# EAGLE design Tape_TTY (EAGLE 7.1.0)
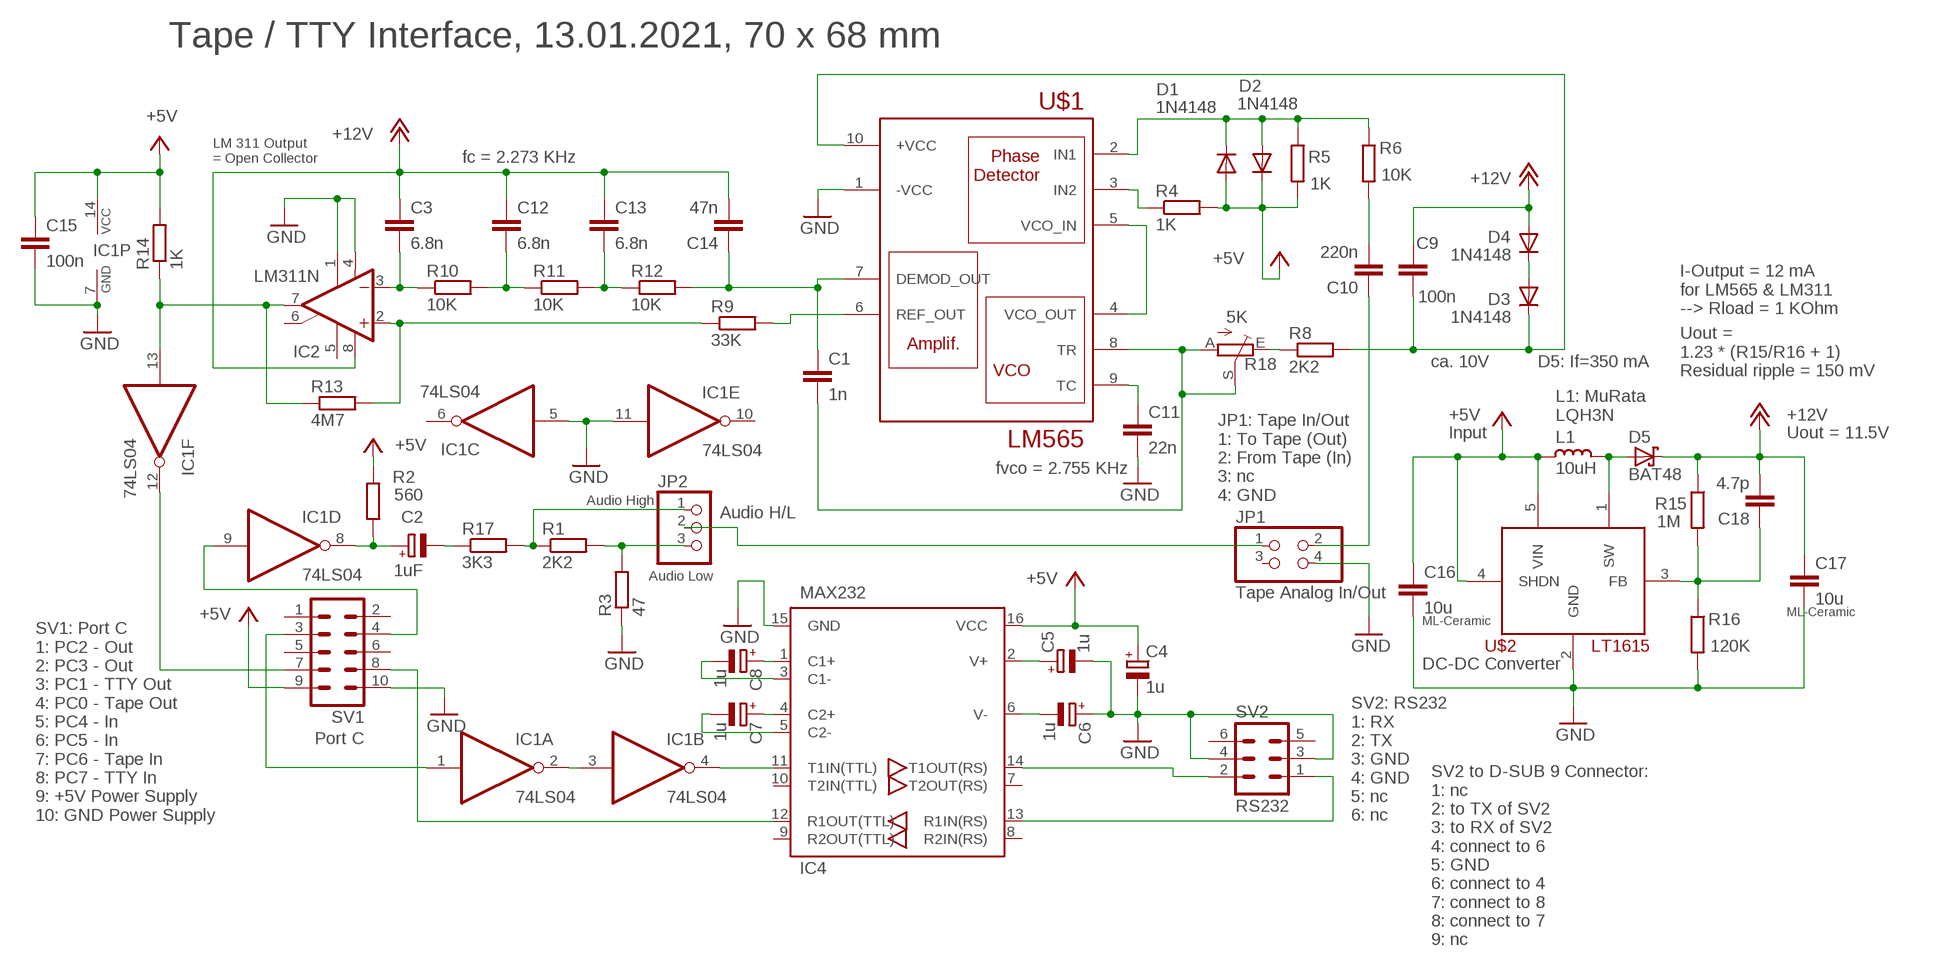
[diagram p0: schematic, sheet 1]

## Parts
C1  1n  C-EUC1206  [C1206]
C2  1uF  CPOL-EUE2-5  [E2-5]
C3  6.8n  C-EU025-025X050  [C025-025X050]
C4  1u  CPOL-EUE2.5-5  [E2,5-5]
C5  1u  CPOL-EUE2.5-5  [E2,5-5]
C6  1u  CPOL-EUE2.5-5  [E2,5-5]
C7  1u  CPOL-EUE2.5-5  [E2,5-5]
C8  1u  CPOL-EUE2.5-5  [E2,5-5]
C9  100n  C-EUC1206  [C1206]
C10  220n  C-EUC1206  [C1206]
C11  22n  C-EUC1206  [C1206]
C12  6.8n  C-EU025-025X050  [C025-025X050]
C13  6.8n  C-EU025-025X050  [C025-025X050]
C14  47n  C-EUC1206  [C1206]
C15  100n  C-EUC1206  [C1206]
C16  10u  C-EUC1210  [C1210]
C17  10u  C-EUC1210  [C1210]
C18  4.7p  C-EUC1206  [C1206]
D1  1N4148  [DO35-10]
D2  1N4148  [DO35-10]
D3  1N4148  [DO35-10]
D4  1N4148  [DO35-10]
D5  BAT48  BAT60J  [SOD323_ST]
IC1  74LS04  7404N  [DIL14]
IC2  LM311N  [DIL08]
IC4  MAX232-1  [DIL16]
JP1  Tape Analog In/Out  PINHD-2X2  [2X02]
JP2  Audio H/L  PINHD-1X3  [1X03]
L1  10uH  L_1206  [L1206]
R1  2K2  R-EU_R1206  [R1206]
R2  560  R-EU_R1206  [R1206]
R3  47  R-EU_R1206  [R1206]
R4  1K  R-EU_R1206  [R1206]
R5  1K  R-EU_R1206  [R1206]
R6  10K  R-EU_R1206  [R1206]
R8  2K2  R-EU_R1206  [R1206]
R9  33K  R-EU_R1206  [R1206]
R10  10K  R-EU_R1206  [R1206]
R11  10K  R-EU_R1206  [R1206]
R12  10K  R-EU_R1206  [R1206]
R13  4M7  R-EU_R1206  [R1206]
R14  1K  R-EU_R1206  [R1206]
R15  1M  R-EU_R1206  [R1206]
R16  120K  R-EU_R1206  [R1206]
R17  3K3  R-EU_R1206  [R1206]
R18  5K  TRIM_EU-CA6V  [CA6V]
SV1  Port C  ML10  [ML10]
SV2  RS232  ML6  [ML6]
U$1  LM565  [DIL14]
U$2  LT1615  [SOT-5-PIN]

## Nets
+5V: C4.+ C15.1 C16.1 D1.A D2.C IC1.14(P:VCC) IC4.16(VCC) L1.2 R2.1 R4.2 R5.2 R14.2 SV1.9 U$2.4(SHDN) U$2.5(VIN)
+12V: C3.1 C9.1 C12.1 C13.1 C14.2 C17.1 C18.2 D4.A D5.C IC2.8(V+) R15.1
GND: C4.- C5.- C6.+ C11.2 C15.2 C16.2 C17.2 IC1.5(C:I) IC1.7(P:GND) IC1.11(E:I) IC2.1(GND) IC2.4(V-) IC4.15(GND) JP1.4 R3.1 R16.2 SV1.10 SV2.3 SV2.4 U$1.1(-VCC) U$2.2(GND)
N$1: IC1.2(A:O) IC1.3(B:I)
N$2: IC1.4(B:O) IC4.11(T1IN(TTL))
N$3: IC1.1(A:I) SV1.3
N$4: IC1.9(D:I) SV1.4
N$5: JP1.1 JP2.2
N$6: C2.+ IC1.8(D:O) R2.2
N$7: C2.- R17.1
N$8: JP2.3 R1.2 R3.2
N$9: R4.1 U$1.3(IN2)
N$10: C1.1 C14.1 R12.2 U$1.7(DEMOD_OUT)
N$11: D1.C D2.A R5.1 R6.1 U$1.2(IN1)
N$12: C10.2 R6.2
N$13: C1.2 R18.A R18.S U$1.8(TR)
N$14: R9.2 U$1.6(REF_OUT)
N$15: R8.1 R18.E
N$16: IC1.12(F:O) SV1.7
N$17: C9.2 D3.C R8.2 U$1.10(+VCC)
N$18: JP2.1 R1.1 R17.2
N$19: IC2.2(+IN) R9.1 R13.2
N$20: IC1.13(F:I) IC2.7(OUT) R13.1 R14.1
N$21: C11.1 U$1.9(TC)
N$22: U$1.4(VCO_OUT) U$1.5(VCO_IN)
N$23: C13.2 R11.2 R12.1
N$24: IC4.12(R1OUT(TTL)) SV1.8
N$25: C8.+ IC4.1(C1+)
N$26: C8.- IC4.3(C1-)
N$27: C6.- IC4.6(V-)
N$28: C7.+ IC4.4(C2+)
N$29: C7.- IC4.5(C2-)
N$30: C5.+ IC4.2(V+)
N$31: C12.2 R10.2 R11.1
N$32: C3.2 IC2.3(-IN) R10.1
N$33: C10.1 JP1.2
N$34: D5.A L1.1 U$2.1(SW)
N$36: D3.A D4.C
N$38: IC4.14(T1OUT(RS)) SV2.2
N$40: C18.1 R15.2 R16.1 U$2.3(FB)
N$42: IC4.13(R1IN(RS)) SV2.1
Unconnected: IC1.6(C:O) IC1.10(E:O) IC2.5(ON) IC2.6(ON/STR) IC4.7(T2OUT(RS)) IC4.8(R2IN(RS)) IC4.9(R2OUT(TTL)) IC4.10(T2IN(TTL)) JP1.3 SV1.1 SV1.2 SV1.5 SV1.6 SV2.5 SV2.6

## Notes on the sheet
- Tape / TTY Interface, 13.01.2021, 70 x 68 mm
- LM 311 Output
  = Open Collector
- fc = 2.273 KHz
- I-Output = 12 mA
  for LM565 & LM311
  --> Rload = 1 KOhm
- ca. 10V | D5: If=350 mA
- Uout =
  1.23 * (R15/R16 + 1)
  Residual ripple = 150 mV
- L1: MuRata
  LQH3N
- Input | Uout = 11.5V
- fvco = 2.755 KHz
- JP1: Tape In/Out
  1: To Tape (Out)
  2: From Tape (In)
  3: nc
  4: GND
- Audio High
- Audio Low
- ML-Ceramic
- ML-Ceramic
- DC-DC Converter
- SV1: Port C
  1: PC2 - Out
  2: PC3 - Out
  3: PC1 - TTY Out
  4: PC0 - Tape Out
  5: PC4 - In
  6: PC5 - In
  7: PC6 - Tape In
  8: PC7 - TTY In
  9: +5V Power Supply
  10: GND Power Supply
- SV2: RS232
  1: RX
  2: TX
  3: GND
  4: GND
  5: nc
  6: nc
- SV2 to D-SUB 9 Connector:
  1: nc
  2: to TX of SV2
  3: to RX of SV2
  4: connect to 6
  5: GND
  6: connect to 4
  7: connect to 8
  8: connect to 7
  9: nc

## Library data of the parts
C1 C3 C9-C18 = rcl:C-EU: CAPACITOR, European symbol
C2 C4-C8 = rcl:CPOL-EU: POLARIZED CAPACITOR, European symbol
D1-D4 = 11manni:1N4148: DIODE
D5 = diode:BAT60J: Schottky barrier diode
IC1 = 74xx-eu:74*04: Hex INVERTER
IC2 = linear3:LM311: COMPARATOR
IC4 = 11manni:MAX232-1
JP1 = 11manni:PINHD-2X2: PIN HEADER
JP2 = 11manni:PINHD-1X3: PIN HEADER
L1 = rc-master-smd:L_: INDUCTOR
R1-R6 R8-R17 = rcl:R-EU_: RESISTOR, European symbol
R18 = 11manni:TRIM_EU-: POTENTIOMETER
SV1 = con-harting-ml:ML10: HARTING; OC_FARNELL: unknown; OC_NEWARK: unknown
SV2 = con-harting-ml:ML6: HARTING; OC_FARNELL: unknown; OC_NEWARK: unknown
U$1 = 11manni:LM565
U$2 = 11manni:LT1615

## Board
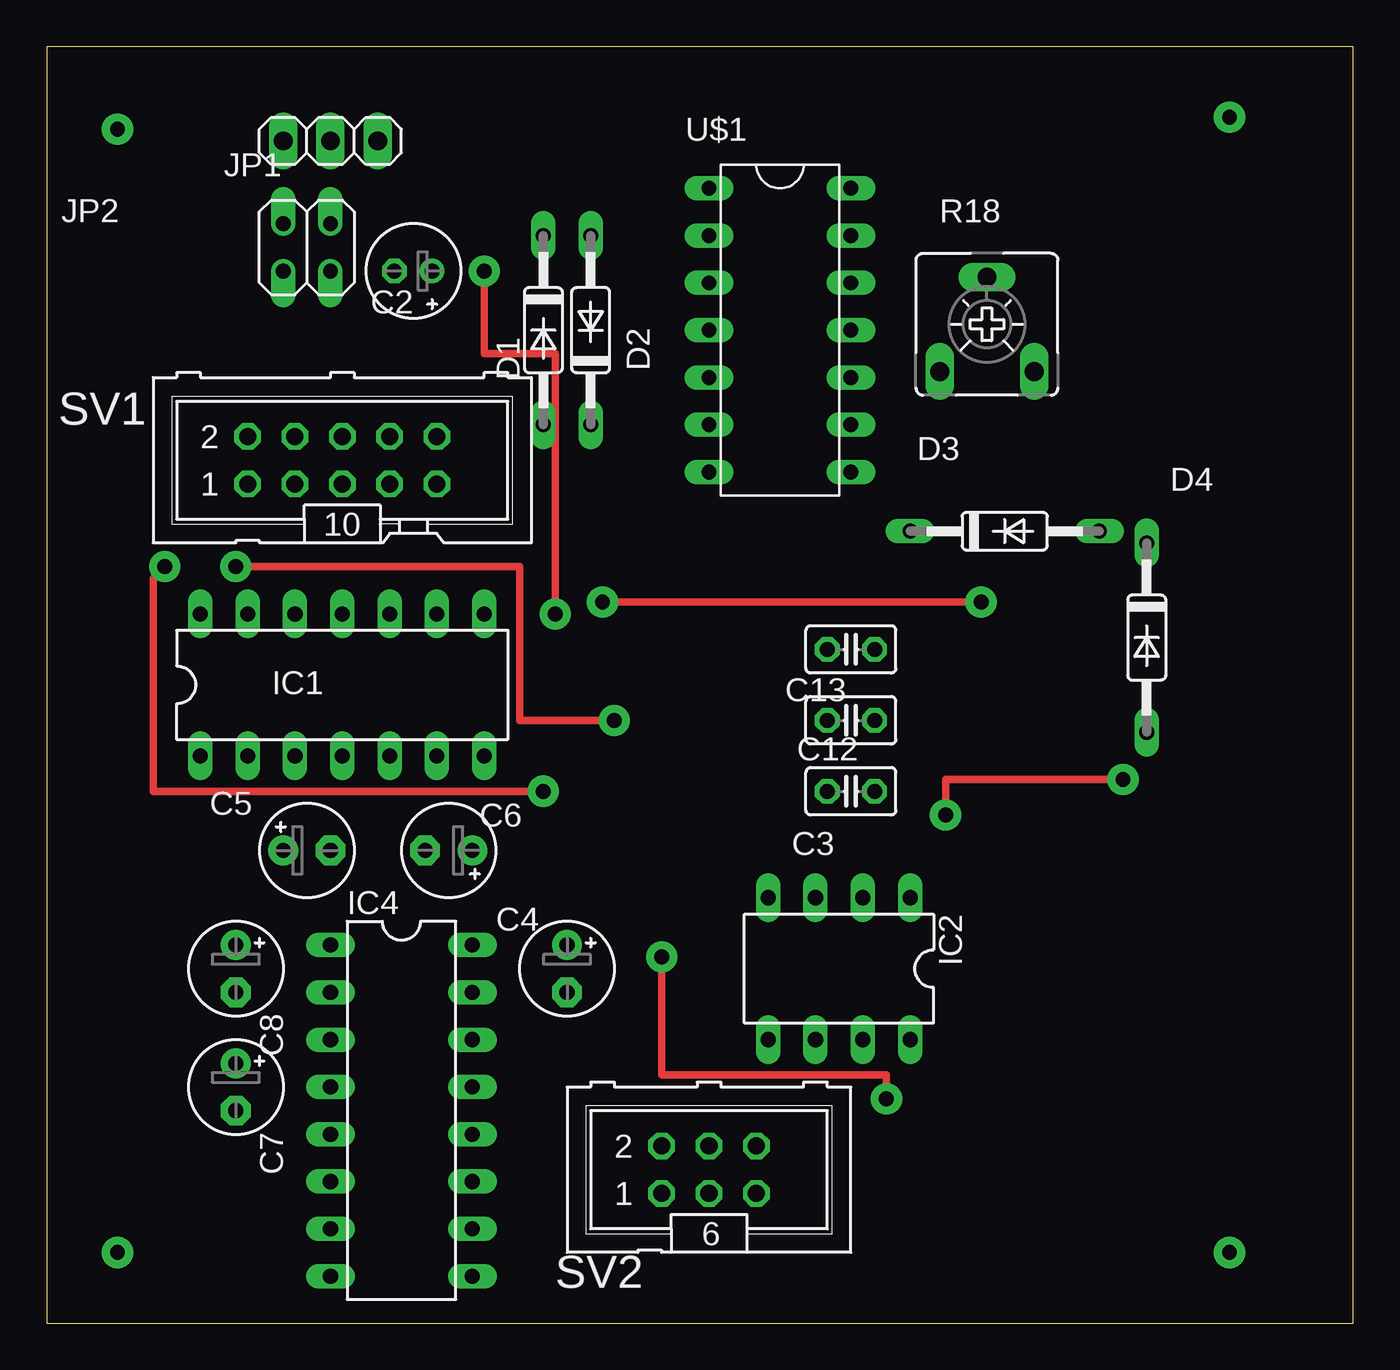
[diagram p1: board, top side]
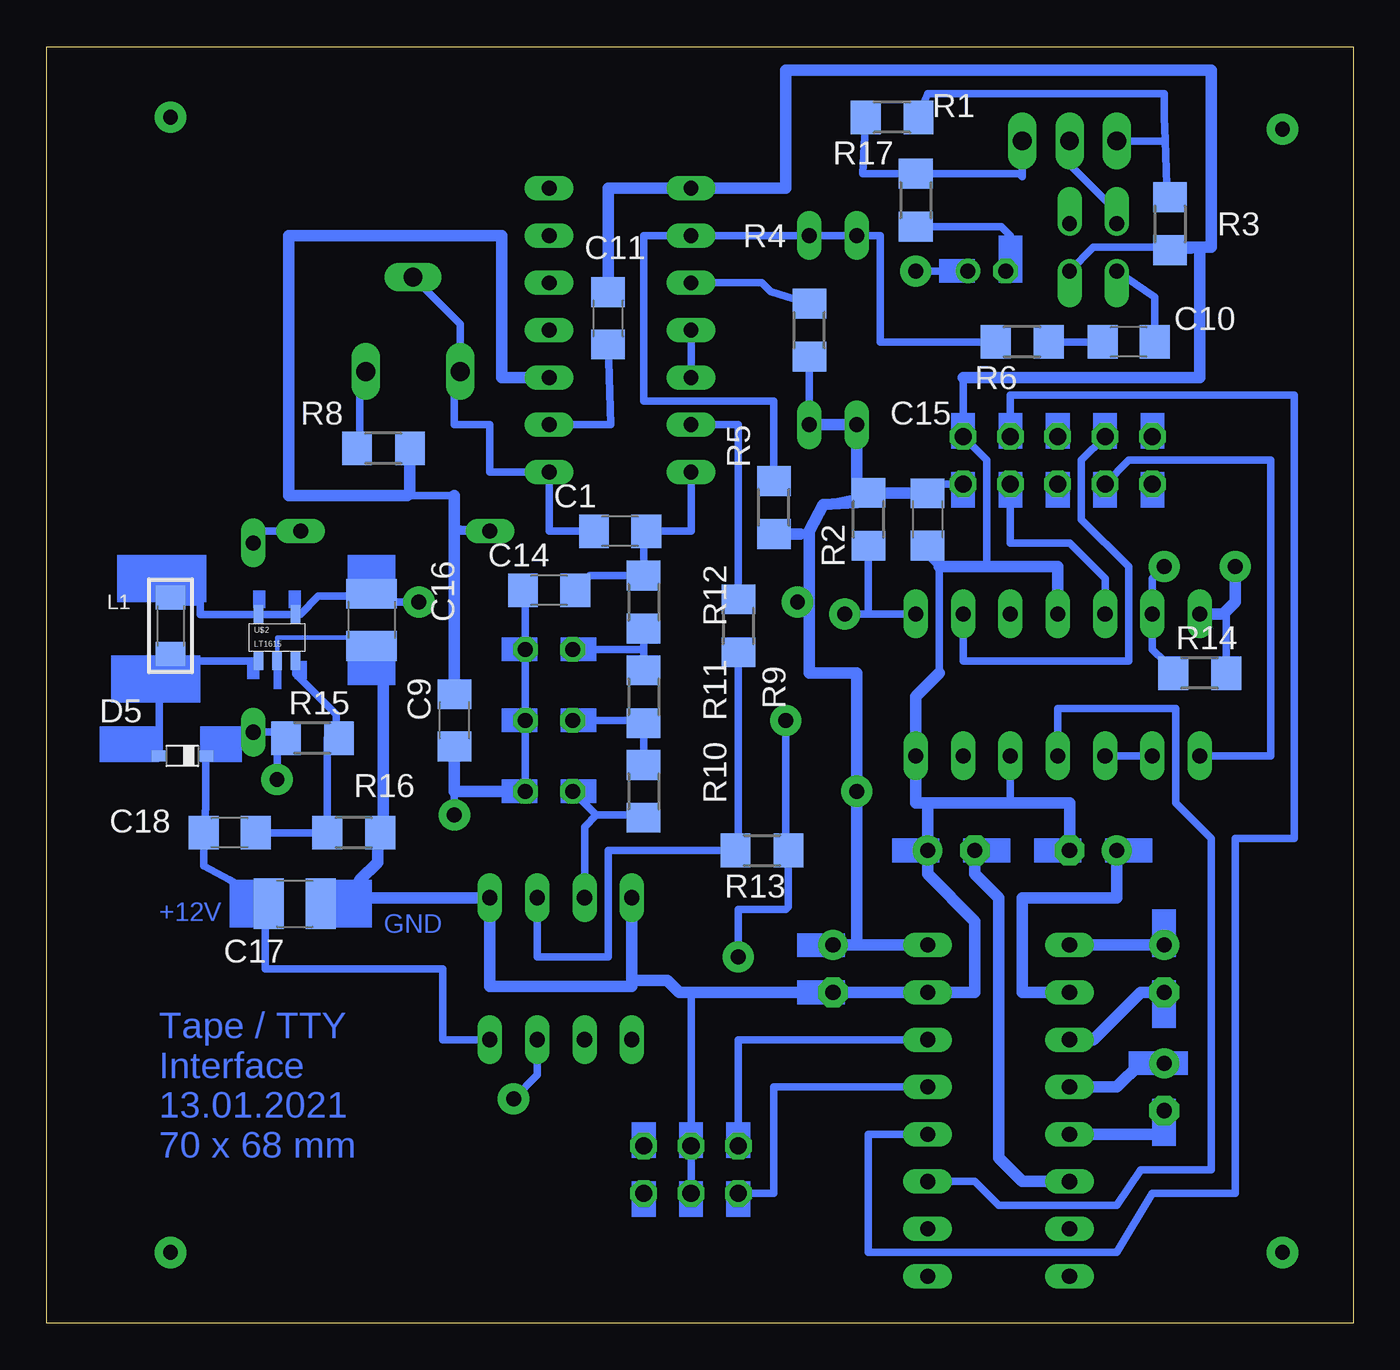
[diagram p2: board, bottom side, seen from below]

Size 70.16 x 68.57 mm. Coordinates in mm from the lower left corner, seen from the top.
Outline: 0,0 70.16,0 70.16,68.57 0,68.57 0,0
Copper layers (1*16): Top 0.035mm / dielectric 1.5mm / Bottom 0.035mm
Design rules "default": minimum track width 10mil, minimum drill 24mil, track to track 8mil, track to pad 8mil, pad to pad 8mil, via to via 8mil, smd to smd 8mil, copper to edge 40mil, drill to drill 8mil, minimum pad ring 10mil, minimum via ring 8mil, stop-mask expansion 4mil, vias tented up to drill 0mil, thermal gap 10mil

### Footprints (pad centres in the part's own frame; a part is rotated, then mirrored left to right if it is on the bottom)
C1206 = smd 1.6 x 1.8: 1 -1.4,0; 2 1.4,0
E2-5 = drill 0.813 pad 1.27: + -1.016,0 | drill 0.813 pad 1.27 octagon: - 1.016,0
C025-025X050 = drill 0.813 octagon: 1 -1.27,0; 2 1.27,0
E2,5-5 = drill 0.813 pad 1.6: + -1.27,0 | drill 0.813 pad 1.6 octagon: - 1.27,0
C1210 = smd 1.6 x 2.7: 1 -1.4,0; 2 1.4,0
DO35-10 = drill 0.813 long: A 5.08,0; C -5.08,0
SOD323_ST = smd 0.8 x 0.6: A 1.25,0; C -1.25,0
DIL14 = drill 0.813 long: 1 -7.62,-3.81; 2 -5.08,-3.81; 3 -2.54,-3.81; 4 0,-3.81; 5 2.54,-3.81; 6 5.08,-3.81; 7 7.62,-3.81; 8 7.62,3.81; 9 5.08,3.81; 10 2.54,3.81; 11 0,3.81; 12 -2.54,3.81; 13 -5.08,3.81; 14 -7.62,3.81
DIL08 = drill 0.813 long: 1 -3.81,-3.81; 2 -1.27,-3.81; 3 1.27,-3.81; 4 3.81,-3.81; 5 3.81,3.81; 6 1.27,3.81; 7 -1.27,3.81; 8 -3.81,3.81
DIL16 = drill 0.813 long: 1 -8.89,-3.81; 2 -6.35,-3.81; 3 -3.81,-3.81; 4 -1.27,-3.81; 5 1.27,-3.81; 6 3.81,-3.81; 7 6.35,-3.81; 8 8.89,-3.81; 9 8.89,3.81; 10 6.35,3.81; 11 3.81,3.81; 12 1.27,3.81; 13 -1.27,3.81; 14 -3.81,3.81; 15 -6.35,3.81; 16 -8.89,3.81
2X02 = drill 0.8 offset: 1 -1.27,1.27; 2 -1.27,-1.27; 3 1.27,1.27; 4 1.27,-1.27
1X03 = drill 1.016 long: 1 -2.54,0; 2 0,0; 3 2.54,0
L1206 = smd 1.3 x 1.6: 1 -1.524,0; 2 1.524,0
R1206 = smd 1.6 x 1.803: 1 -1.422,0; 2 1.422,0
CA6V = drill 1.016 long: A -2.54,-2.54; E 2.54,-2.54; S 0,2.54
ML10 = drill 0.914 octagon: 1 -5.08,-1.27; 2 -5.08,1.27; 3 -2.54,-1.27; 4 -2.54,1.27; 5 0,-1.27; 6 0,1.27; 7 2.54,-1.27; 8 2.54,1.27; 9 5.08,-1.27; 10 5.08,1.27
ML6 = drill 0.914 octagon: 1 -2.54,-1.27; 2 -2.54,1.27; 3 0,-1.27; 4 0,1.27; 5 2.54,-1.27; 6 2.54,1.27
DIL14' = drill 0.8 long: 1 -3.81,7.62; 2 -3.81,5.08; 3 -3.81,2.54; 4 -3.81,0; 5 -3.81,-2.54; 6 -3.81,-5.08; 7 -3.81,-7.62; 8 3.81,-7.62; 9 3.81,-5.08; 10 3.81,-2.54; 11 3.81,0; 12 3.81,2.54; 13 3.81,5.08; 14 3.81,7.62
SOT-5-PIN = smd 0.5 x 1: 1 -1,-1.25; 2 0,-1.25; 3 1,-1.25; 4 1,1.25; 5 -1,1.25

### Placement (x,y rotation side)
C1  39.37,42.55 180 bottom
C2  19.68,56.52 180 top
C3  43.18,28.57 180 top
C4  27.94,19.05 270 top
C5  13.97,25.4 0 top
C6  21.59,25.4 180 top
C7  10.16,12.7 270 top
C8  10.16,19.05 270 top
C9  48.26,32.38 90 bottom
C10  12.06,52.7 180 bottom
C11  40.01,53.98 90 bottom
C12  43.18,32.38 180 top
C13  43.18,36.2 180 top
C14  43.18,39.37 180 bottom
C15  22.86,43.18 270 bottom
C16  52.7,37.78 270 bottom
C17  56.83,22.54 0 bottom
C18  60.33,26.35 180 bottom
D1  26.67,53.34 270 top
D2  29.21,53.34 90 top
D3  51.44,42.55 0 top
D4  59.05,36.83 270 top
D5  62.87,30.48 180 bottom
IC1  15.88,34.29 0 top
IC2  42.55,19.05 180 top
IC4  19.05,11.43 270 top
JP1  13.97,57.78 0 top
JP2  15.24,63.5 180 top
L1  63.5,37.47 90 bottom
R1  24.77,64.77 0 bottom
R2  26.04,43.18 270 bottom
R3  9.84,59.05 90 bottom
R4  29.21,53.34 270 bottom
R5  31.11,43.81 270 bottom
R6  17.78,52.7 0 bottom
R8  52.07,46.99 0 bottom
R9  33.02,37.47 90 bottom
R10  38.1,28.57 90 bottom
R11  38.1,33.66 90 bottom
R12  38.1,38.73 90 bottom
R13  31.75,25.4 180 bottom
R14  8.26,34.92 0 bottom
R15  55.88,31.43 0 bottom
R16  53.66,26.35 0 bottom
R17  23.5,60.33 90 bottom
R18  50.48,53.66 0 top
SV1  15.88,46.35 0 top
SV2  35.56,8.26 0 top
U$1  LM565  [DIL14']  39.37,53.34 0 top
U$2  57.78,36.83 0 bottom

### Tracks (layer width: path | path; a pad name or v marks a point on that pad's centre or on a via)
+5V  (via drill 0.8 pad 1.68)
  Top 0.406: v26.67,28.57 5.71,28.57 5.71,40.01 v6.35,40.64 | v50.16,38.73 v29.84,38.73
  Bottom 0.406: 28.47,43.97 26.19,44.45 R2.1 26.01,44.58 | R4.2 D2.C | R14.2 6.83,37.95 6.99,38.1 | 29.69,42.39 29.21,42.55 | v50.16,38.73 52.26,38.73 C16.1 52.84,39.05 55.56,39.05 56.53,38.08 U$2.4 U$2.5 61.91,38.08 61.91,38.73 63.5,38.73 L1.2 | v29.84,38.73 29.21,38.73 | SV1.9 22.36,45.09 C15.1
  Bottom 0.61: C4.+ 26.67,20.32 | 26.67,20.32 IC4.16 | 26.67,20.32 v26.67,28.57 26.67,34.92 29.21,34.92 29.21,38.73 29.21,42.55 28.47,43.97 26.67,44.07 D1.A D2.C | v6.35,40.64 6.35,38.73 6.99,38.1 IC1.14 | R5.2 29.69,42.39 | C15.1 26.01,44.58
+12V  (via drill 0.8 pad 1.68)
  Top 0.406: v57.78,29.21 48.26,29.21 v48.26,27.3
  Bottom 0.406: 57.78,31.75 D4.A D5.C 61.62,27.73 C18.2 61.73,24.58 60.33,23.81 C17.1 58.42,22.36 58.42,19.05 48.9,19.05 48.9,15.24 IC2.8 | 57.78,31.75 57.62,31.75 R15.1 | C3.1 C12.1 C13.1 44.45,39.24 C14.2 | v57.78,29.21 57.78,31.75 | 48.26,28.57 v48.26,27.3
  Bottom 0.61: C3.1 48.26,28.57 C9.1
GND
  Bottom 0.254: U$2.2 57.78,36.83 53.15,36.83 C16.2
  Bottom 0.305: 52.7,36.83 52.52,36.51 C16.2 52.7,36.51 | 52.07,27.15 R16.2
  Bottom 0.406: 52.7,36.51 52.07,34.29 | 53.34,23.81 C17.2 55.24,23.62 53.98,22.86 | 52.39,26.84 R16.2 | 22.23,34.92 22.23,40.64 22.86,41.27 C15.2 | 35.56,17.78 SV2.4 SV2.3 | 19.68,40.64 19.68,46.35 SV1.10 20.95,50.8 | JP1.4 13.97,57.78 9.53,57.78 | 8.26,57.78 8.1,57.78 7.77,57.78 R3.1 | IC1.5 18.41,27.94
  Bottom 0.61: C5.- 15.24,27.94 18.41,27.94 22.86,27.94 | 22.86,27.94 C6.+ 22.86,24.13 20.32,21.59 20.32,17.78 IC4.15 C4.- 35.56,17.78 36.2,17.78 36.83,18.41 38.73,18.41 | 52.07,34.29 52.07,27.15 | 53.34,23.81 52.39,24.77 52.39,26.84 | 22.86,27.94 23.5,27.94 IC1.7 23.5,33.66 22.23,34.92 | 22.23,40.64 19.68,40.64 15.88,40.64 IC1.11 | 20.95,50.8 8.26,50.8 8.26,57.78 9.53,57.78 R3.1 8.1,57.78 7.62,57.78 7.62,67.31 30.48,67.31 30.48,60.96 U$1.1 40.01,60.96 C11.2 | IC2.4 38.73,18.41 | 38.73,18.41 38.73,18.1 46.35,18.1 IC2.1 53.98,22.86
N$1
  Bottom 0.406: IC1.2 IC1.3
N$2
  Bottom 0.406: IC1.4 15.88,33.02 9.53,33.02 9.53,27.94 7.62,26.04 7.62,8.26 11.43,8.26 12.7,6.35 19.05,6.35 20.32,7.62 IC4.11
N$3
  Bottom 0.406: SV1.3 12.06,46.35 4.45,46.35 4.45,30.48 IC1.1
N$4
  Bottom 0.406: SV1.4 14.61,46.35 14.61,43.18 12.06,40.64 12.06,35.56 20.95,35.56 IC1.9
N$5
  Bottom 0.406: JP1.1 12.7,59.69 15.24,62.23 JP2.2
N$6  (via drill 0.8 pad 1.68)
  Top 0.406: v23.5,56.52 23.5,52.07 27.3,52.07 v27.3,38.1
  Bottom 0.406: 26.04,41.91 R2.2 26.04,38.1 | 26.04,38.1 IC1.8 | v27.3,38.1 26.04,38.1 | v23.5,56.52 C2.+
N$7
  Bottom 0.406: R17.1 18.9,58.9 18.41,58.42 18.41,56.77 C2.-
N$8
  Bottom 0.406: R1.2 23.34,64.92 22.86,66.04 10.16,66.04 10.16,64.77 10.11,63.53 | R3.2 10.01,61.11 10.11,63.53 | JP2.3 10.11,63.5 10.11,63.53
N$9
  Bottom 0.406: R4.1 31.27,55.4 31.75,55.88 U$1.3
N$10
  Bottom 0.406: U$1.7 35.56,42.55 C1.1 38.1,42.41 R12.2 40.99,40.16 C14.1
N$11
  Bottom 0.406: R6.1 25.4,52.7 25.4,58.42 D1.C D2.A U$1.2 38.1,58.42 38.1,49.53 31.11,49.53 R5.1
N$12
  Bottom 0.406: C10.2 R6.2
N$13
  Bottom 0.406: C1.2 43.18,42.55 U$1.8 46.35,45.72 46.35,48.26 48.26,48.26 48.26,50.8 47.94,50.8 R18.A 47.94,53.66 R18.S 50.65,56.03
N$14
  Bottom 0.406: R9.2 33.02,48.26 U$1.6
N$15
  Bottom 0.406: R8.1 53.34,46.35 53.34,50.8 53.02,50.8 R18.E
N$16
  Bottom 0.406: IC1.12 13.34,40.01 15.24,41.91 18.41,41.91 SV1.7
N$17
  Bottom 0.406: 48.26,42.55 D3.C 48.26,42.7 | 48.26,44.45 50.8,44.45 50.65,44.6
  Bottom 0.61: C9.2 48.26,42.55 | U$1.10 45.72,50.8 45.72,58.42 57.15,58.42 57.15,44.45 50.8,44.45 | 48.26,44.45 48.26,42.7 | R8.2 50.65,44.6
N$18
  Bottom 0.406: R1.1 26.34,61.75 R17.2 17.93,61.75 17.78,61.59 JP2.1
N$19
  Bottom 0.406: R9.1 33.02,25.4 R13.2 40.01,25.4 40.01,19.68 43.81,19.68 IC2.2
N$20  (via drill 0.8 pad 1.68)
  Top 0.406: v33.02,19.68 33.02,13.34 45.09,13.34 v45.09,12.06 | v10.16,40.64 25.4,40.64 25.4,32.38 v30.48,32.38
  Bottom 0.406: R14.1 10.16,35.56 10.79,36.2 IC1.13 10.79,40.01 v10.16,40.64 | v30.48,32.38 30.48,25.55 R13.1 30.33,22.38 30.48,22.23 33.02,22.23 v33.02,19.68 | v45.09,12.06 43.81,13.34 IC2.7
N$21
  Bottom 0.406: U$1.9 39.88,48.26 C11.1
N$22
  Bottom 0.406: U$1.4 U$1.5
N$23
  Bottom 0.406: R12.1 38.1,36.2 | 38.1,36.2 R11.2 | C13.2 38.1,36.2
N$24
  Bottom 0.406: SV1.8 18.41,49.85 3.17,49.85 3.17,26.04 6.35,26.04 6.35,6.99 10.79,6.99 12.7,3.81 26.04,3.81 26.04,10.16 IC4.12
N$25
  Bottom 0.61: IC4.1 C8.+
N$26
  Bottom 0.406: IC4.3 13.97,15.24
  Bottom 0.61: 13.97,15.24 11.43,17.78 C8.-
N$27
  Bottom 0.61: C6.- 20.32,24.13 19.05,22.86 19.05,8.89 17.78,7.62 IC4.6
N$28
  Bottom 0.61: IC4.4 12.7,12.7 11.43,13.97 C7.+
N$29
  Bottom 0.61: IC4.5 10.16,10.16 C7.-
N$30
  Bottom 0.61: IC4.2 17.78,17.78 17.78,22.86 12.7,22.86 C5.+
N$31
  Bottom 0.406: R10.2 R11.1 38.25,32.38 C12.2
N$32
  Bottom 0.406: C3.2 40.64,27.3 | 40.64,27.3 38.25,27.3 R10.1 | IC2.3 41.27,26.67 40.64,27.3
N$33
  Bottom 0.406: C10.1 10.66,55.12 JP1.2
N$34
  Bottom 0.406: D5.A 64.11,34.27 64.14,34.29 63.48,34.63 62.87,35.24 | 62.87,35.24 63.56,35.24 L1.1 | U$2.1 60.62,35.58 60.64,35.56 62.55,35.56 62.87,35.24
N$36
  Bottom 0.406: D3.A 59.05,42.55 D4.C
N$38
  Bottom 0.406: IC4.14 33.02,15.24 SV2.2
N$40
  Bottom 0.406: C18.1 R16.1 55.08,31.45 R15.2 54.61,32.22 54.61,32.7 56.78,34.88 U$2.3
N$42
  Bottom 0.406: IC4.13 31.11,12.7 31.11,6.99 SV2.1
N$49  (via drill 0.8 pad 1.68)
  other vias: 3.81,64.14
N$51  (via drill 0.8 pad 1.68)
  other vias: 63.5,64.77
N$52  (via drill 0.8 pad 1.68)
  other vias: 63.5,3.81
N$53  (via drill 0.8 pad 1.68)
  other vias: 3.81,3.81
(copper drawn outside any net)
  shapes: Bottom area x49

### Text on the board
Bottom: +12V | GND | Tape / TTY / Interface / 13.01.2021 / 70 x 68 mm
